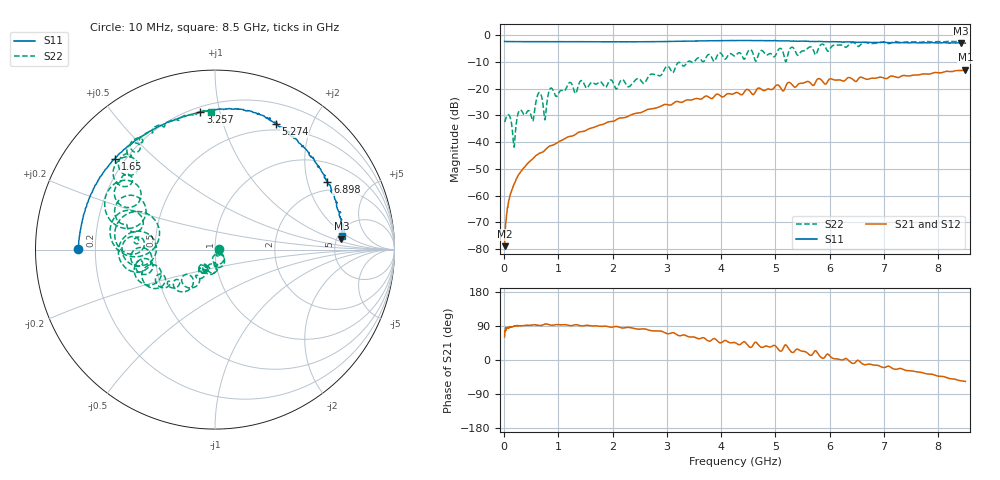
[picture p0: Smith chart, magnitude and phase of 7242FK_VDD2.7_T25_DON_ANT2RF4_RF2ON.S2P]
!Agilent Technologies,E5071C,MY46417908,A.11.23
!Date: Wed Dec 09 15:39:23 2020
!Data & Calibration Information:
!Freq	S11:SOLT2(ON)	S21:SOLT2(ON)	S12:SOLT2(ON)	S22:SOLT2(ON)
!PortZ  Port1:50+j0  Port2:50+j0
!Above PortZ is port z conversion or system Z0 setting when saving the data.
!When reading, reference impedance value at option line is always used.
# Hz S dB R 50
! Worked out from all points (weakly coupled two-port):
!   1601 points, 10 MHz to 8.5 GHz, reference 50 ohm
!   highest |S21| = -12.93 dB at 8.5 GHz (marker M1); lowest = -78.9 dB at 10 MHz (marker M2)
!   lowest |S11| = -3.0 dB at 8.42 GHz (marker M3), VSWR 5.83, Z = 275 + j67 ohm
!   |S11| at or under -10 dB: nowhere
!   |S22| runs from -41.9 to -2.2 dB; largest |S21 - S12| = 0.0033
!   S11 on the Smith chart (normalised r, x): 10 MHz: 0.13, +0.00; 1.65 GHz: 0.16, +0.38; 3.257 GHz: 0.23, +0.87; 5.274 GHz: 0.43, +1.51; 6.898 GHz: 1.65, +2.68; 8.5 GHz: 5.36, +1.65
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1e7  -2.34 179.7  -78.87 60.8  -78.68 69.6  -32.46 2.6
8.42875e7  -2.38 177.5  -61.96 84.7  -62.34 84.7  -29.74 -33.5
1.851062e8  -2.40 174.6  -55.70 90.0  -55.65 89.8  -41.87 -30.3
3.018438e8  -2.42 171.4  -51.19 90.1  -51.14 89.7  -27.93 -44.0
5.247062e8  -2.41 165.4  -46.25 92.3  -46.26 92.5  -32.07 -59.7
6.520562e8  -2.42 162.2  -44.13 91.2  -44.12 91.2  -21.43 -72.3
7.52875e8  -2.43 159.6  -43.00 94.7  -43.02 94.7  -31.65 -72.1
8.59e8  -2.42 156.8  -41.30 92.1  -41.30 92.1  -19.81 -71.2
1.426769e9  -2.43 143.5  -36.04 89.9  -36.05 89.8  -16.95 -105.0
1.649631e9  -2.47 137.7  -34.49 89.9  -34.50 89.9  -17.91 -115.0
2.843538e9  -2.40 105.8  -26.94 76.5  -26.95 76.5  -15.08 -125.7
3.257425e9  -2.24 96.0  -25.12 64.3  -25.12 64.3  -10.56 -141.5
4.255e9  -2.02 77.6  -21.61 45.8  -21.61 45.8  -7.72 -168.9
5.077469e9  -2.14 65.7  -19.10 24.5  -19.07 24.4  -4.98 172.3
5.1889e9  -2.17 63.7  -19.12 40.1  -19.13 39.9  -9.94 166.5
5.2738e9  -2.20 64.2  -17.84 24.0  -17.80 24.0  -4.88 176.5
5.671769e9  -2.33 54.9  -18.50 13.3  -18.45 13.2  -4.65 149.7
5.777894e9  -2.34 54.4  -16.33 18.4  -16.33 18.5  -5.70 166.8
6.897512e9  -2.71 31.1  -15.76 -14.7  -15.79 -14.6  -2.93 132.6
7.088538e9  -2.78 27.0  -15.69 -16.4  -15.75 -16.3  -3.17 127.6
8.420406e9  -3.01 4.9  -13.22 -54.9  -13.30 -55.2  -2.22 94.2
8.5e9  -2.98 6.2  -12.93 -56.7  -13.03 -56.6  -2.30 91.5
